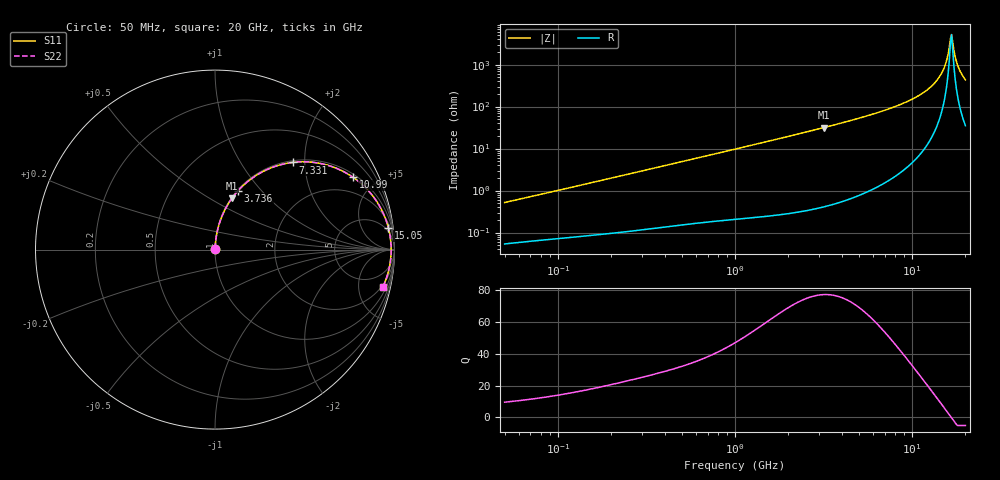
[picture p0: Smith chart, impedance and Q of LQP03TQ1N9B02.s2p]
!Murata Part Number: LQP03TQ1N9B02
!These Parameters are Measured in Series Mode Connection
!  o--[Z]--o
!Port1  Port2
!  o-------o
!Freq. Start=50[MHz] Stop=20[GHz], 401[Steps]
# Hz S RI R 50
!Freq.(Hz) S11(Real) S11(Imag) S21(Real) S21(Imag) S12(Real) S12(Imag) S22(Real) S22(Imag)
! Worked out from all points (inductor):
!   401 points, 50 MHz to 20 GHz, reference 50 ohm
!   read as one part in series: L = 1.63 nH near 51.52 MHz
!   highest Q = 77.2 at 3.169 GHz (marker M1), where L = 1.59 nH
!   self-resonance near 16.46 GHz
!   S11 on the Smith chart (normalised r, x): 50 MHz: 1.00, +0.01; 3.736 GHz: 1.01, +0.76; 7.331 GHz: 1.03, +1.74; 10.99 GHz: 1.14, +3.72; 15.05 GHz: 3, +15; 20 GHz: 1.70, -8.67
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5e7  0.000563 0.00516  0.9994 -0.00516  0.9994 -0.00516  0.000563 0.00516
1.364002e8  0.000998 0.0136  0.999 -0.0136  0.999 -0.0136  0.000998 0.0136
3.721004e8  0.00262 0.0363  0.9974 -0.0363  0.9974 -0.0363  0.00262 0.0363
1e9  0.0113 0.0956  0.9887 -0.0956  0.9887 -0.0956  0.0113 0.0956
2.728004e9  0.0704 0.2494  0.9296 -0.2494  0.9296 -0.2494  0.0704 0.2494
3.168813e9  0.0937 0.285  0.9063 -0.285  0.9063 -0.285  0.0937 0.285
3.736399e9  0.1281 0.3277  0.8719 -0.3277  0.8719 -0.3277  0.1281 0.3277
5.352748e9  0.2504 0.4258  0.7496 -0.4258  0.7496 -0.4258  0.2504 0.4258
7.331367e9  0.4335 0.4859  0.5665 -0.4859  0.5665 -0.4859  0.4335 0.4859
7.442007e9  0.4443 0.487  0.5557 -0.487  0.5557 -0.487  0.4443 0.487
1.098561e10  0.7681 0.4039  0.2319 -0.4039  0.2319 -0.4039  0.7681 0.4039
1.334722e10  0.9122 0.2505  0.0878 -0.2505  0.0878 -0.2505  0.9122 0.2505
1.438523e10  0.95 0.1721  0.05 -0.1721  0.05 -0.1721  0.95 0.1721
1.504638e10  0.966 0.1214  0.034 -0.1214  0.034 -0.1214  0.966 0.1214
1.573793e10  0.9765 0.0687  0.0235 -0.0687  0.0235 -0.0687  0.9765 0.0687
1.621653e10  0.9803 0.0329  0.0197 -0.0329  0.0197 -0.0329  0.9803 0.0329
1.670968e10  0.9815 -0.00313  0.0185 0.00313  0.0185 0.00313  0.9815 -0.00313
1.696185e10  0.981 -0.0212  0.019 0.0212  0.019 0.0212  0.981 -0.0212
1.774144e10  0.9758 -0.0749  0.0242 0.0749  0.0242 0.0749  0.9758 -0.0749
1.828096e10  0.9691 -0.1101  0.0309 0.1101  0.0309 0.1101  0.9691 -0.1101
1.912117e10  0.9543 -0.1615  0.0457 0.1615  0.0457 0.1615  0.9543 -0.1615
2e10  0.9344 -0.2103  0.0656 0.2103  0.0656 0.2103  0.9344 -0.2103
